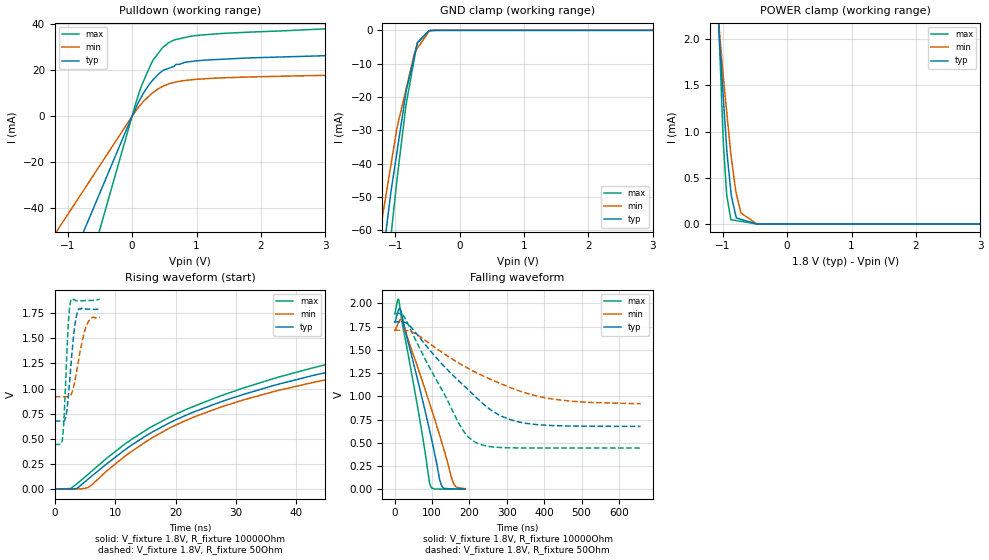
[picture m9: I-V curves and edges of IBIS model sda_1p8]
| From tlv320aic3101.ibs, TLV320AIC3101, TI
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|   sda_1p8 Model
[Model]   sda_1p8
Model_type   I/O_open_drain
Polarity   Inverting
Vinl = 0.54
Vinh = 1.26
Vmeas = 0.9
Vref = 1.8
Cref = 2pF
Rref = 10000
|   typ   min   max
|   (nom PVT)   (fast PVT)   (slow PVT)
 C_comp   1.241e-12   1.230e-12   1.247e-12
| Where nom  PVT is Nominal Process, 1.8V, 27C
|   Fast PVT is Strong Process,  1.89V, -40C
|   Slow PVT is Weak Process,   1.71V, 105C
[Model Spec]
|Subparameter   typ   min   max
Vinh   1.26   1.197   1.323
Vinl   0.54   0.513   0.567
[Voltage Range]   1.8   1.71   1.89
|Ambient Temperature   25   85   -40
|Junction Temperature
[Temperature Range]   27   105   -40
[Pullup Reference]   1.8   1.71   1.89
[Pulldown Reference]   0   0   0
[Power Clamp Reference]   1.8   1.71   1.89
[GND Clamp Reference]   0   0   0
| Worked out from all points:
|   slope of the pulldown table from 0 to 0.27 V, typ, clamps not added: 19.4 ohm
|   GND clamp passes 1 mA (typ) near -0.52 V on its own axis
|   POWER clamp passes 1 mA (typ) near -0.96 V on its own axis
|   falling waveform, V_fixture 1.8V, R_fixture 10000Ohm: 20-80 % time 62.9ns typ, 80.6ns min, 48.8ns max; typ from 1.8 V to 0.003 V
|   rising waveform, V_fixture 1.8V, R_fixture 10000Ohm: 20-80 % time 62.1ns typ, 64.7ns min, 60.1ns max; typ from 0.003 V to 1.8 V
|   falling waveform, V_fixture 1.8V, R_fixture 50Ohm: 20-80 % time 164ns typ, 221ns min, 112ns max; typ from 1.8 V to 0.677 V
|   rising waveform, V_fixture 1.8V, R_fixture 50Ohm: 20-80 % time 989ps typ, 1.52ns min, 643ps max; typ from 0.677 V to 1.79 V
[Pulldown]
|   Voltage   I(typ)   I(min)   I(max)
-1.8V     -119.7mA   -76.78mA   -176.3mA
-66.6mV   -4.429mA   -2.841mA   -6.521mA
51.03mV   3.137mA    2.019mA    5.146mA
145.5mV   8.419mA    5.427mA    13.24mA
302.4mV   15.09mA    9.788mA    23.13mA
470.6mV   19.63mA    12.87mA    29.69mA
574.6mV   20.84mA    14.08mA    31.98mA
655.8mV   21.67mA    14.68mA    33.06mA
677.4mV   22.45mA    14.8mA     33.2mA
817.2mV   23.33mA    15.48mA    34.09mA
1.139V    24.33mA    16.25mA    35.33mA
3.6V      26.81mA    18.04mA    38.66mA
[GND Clamp]
|   Voltage   I(typ)   I(min)   I(max)
-1.8V     -219.5mA   -139.2mA   -296mA
-1.375V   -96.64mA   -76.85mA   -123.8mA
-1.092V   -52.6mA    -43.52mA   -66.66mA
-1.067V   -48.7mA    -40.57mA   -62.12mA
-969.6mV  -36.18mA   -29.07mA   -44.35mA
-831.6mV  -18.52mA   -17.67mA   -22.39mA
-696mV    -7.282mA   -6.465mA   -7.757mA
-659.6mV  -4.308mA   -5.458mA   -3.835mA
-651.6mV  -3.652mA   -5.237mA   -3.674mA
-470.6mV  -85.43uA   -227.4uA   -29.15uA
-289mV    -542.8nA   -2.787uA   -121.7nA
3.6V      0A         0A         0A
[POWER Clamp]
|   Voltage   I(typ)   I(min)   I(max)
-1.8V     11.74mA    8.633mA    19.35mA
-1.081V   2.386mA    2.338mA    2.535mA
-1.04V    1.89mA     2.005mA    1.793mA
-990.4mV  1.367mA    1.596mA    886.6uA
-937.4mV  814.2uA    1.215mA    315.3uA
-930.6mV  748.9uA    1.166mA    286.6uA
-873.2mV  356.4uA    756.1uA    45.76uA
-865.8mV  305.9uA    716.4uA    44.92uA
-788.4mV  64.55uA    328.2uA    36.12uA
-714.8mV  49.55uA    117.7uA    27.76uA
-470.3mV  0A         257nA      0A
3.6V      0A         0A         0A
[Ramp]
R_load = 10000
|   typ   min   max
dV/dt_r   1.07817/6.1534e-08   1.02313/6.43248e-08   1.1328/5.95906e-08
dV/dt_f   1.07839/6.29157e-08   1.02357/8.06665e-08   1.13293/4.88677e-08
[Falling Waveform]
V_fixture = 1.8V
V_fixture_min = 1.71V
V_fixture_max = 1.89V
R_fixture = 10000Ohm
|   Time   V(typ)   V(min)   V(max)
0s        1.8V       1.71V      1.89V
8.425ns   1.904V     1.775V     2.04V
11.6ns    1.939V     1.804V     2.03V
16.6ns    1.926V     1.828V     1.892V
22.45ns   1.822V     1.796V     1.743V
67.83ns   1.075V     1.241V     741mV
95.42ns   602.9mV    902.9mV    42.91mV
125.2ns   44.72mV    518.8mV    2.511mV
157.9ns   4.33mV     63.59mV    1.9mV
188.4ns   2.992mV    7.005mV    1.792mV
[Rising Waveform]
V_fixture = 1.8V
V_fixture_min = 1.71V
V_fixture_max = 1.89V
R_fixture = 10000Ohm
|   Time   V(typ)   V(min)   V(max)
0s        2.687mV    4.034mV    1.775mV
2.65ns    502.5uV    3.691mV    6.682mV
5.475ns   98.86mV    16.5mV     145.5mV
16.2ns    570.7mV    514.3mV    627mV
31.4ns    945.4mV    890.6mV    1.009V
56ns      1.293V     1.208V     1.38V
79.65ns   1.49V      1.389V     1.587V
113.1ns   1.646V     1.539V     1.746V
155.1ns   1.736V     1.633V     1.834V
278.1ns   1.8V       1.71V      1.89V
[Falling Waveform]
V_fixture = 1.8V
V_fixture_min = 1.71V
V_fixture_max = 1.89V
R_fixture = 50Ohm
|   Time   V(typ)   V(min)   V(max)
0s        1.8V       1.71V      1.89V
25.8ns    1.797V     1.71V      1.855V
57.05ns   1.682V     1.672V     1.599V
175.3ns   1.153V     1.35V      684.9mV
196.8ns   1.072V     1.301V     565.1mV
221ns     977.9mV    1.25V      496.2mV
276.1ns   807.2mV    1.15V      451.5mV
341.5ns   717.1mV    1.048V     444.9mV
473.6ns   680.6mV    947.6mV    444.3mV
658ns     677.4mV    920.3mV    444.3mV
[Rising Waveform]
V_fixture = 1.8V
V_fixture_min = 1.71V
V_fixture_max = 1.89V
R_fixture = 50Ohm
|   Time   V(typ)   V(min)   V(max)
0s        677.4mV    919.8mV    444.3mV
1.025ns   677.4mV    919.8mV    446.3mV
1.325ns   676.6mV    919.9mV    524.6mV
1.825ns   718.9mV    919.5mV    1.096V
2.225ns   911.3mV    918.9mV    1.63V
2.65ns    1.218V     936.1mV    1.876V
3.275ns   1.605V     1.06V      1.884V
3.9ns     1.785V     1.267V     1.873V
5.275ns   1.79V      1.632V     1.875V
7.45ns    1.79V      1.71V      1.89V
